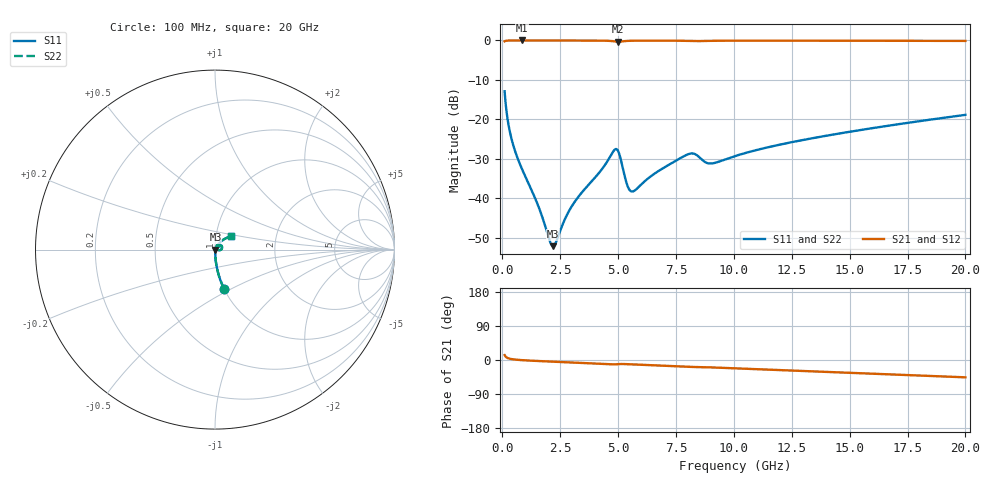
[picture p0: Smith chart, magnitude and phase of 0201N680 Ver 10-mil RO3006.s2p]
# GHz S MA R 50
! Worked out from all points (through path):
!   1601 points, 100 MHz to 20 GHz, reference 50 ohm
!   highest |S21| = -0.02 dB at 833.8 MHz (marker M1); lowest = -0.3 dB at 4.988 GHz (marker M2)
!   group delay of S21, straight-line fit = 6.5 ps
!   lowest |S11| = -52.1 dB at 2.189 GHz (marker M3), VSWR 1.00, Z = 50.2 - j0.0379 ohm
!   |S11| at or under -10 dB: start of sweep to end of sweep
!   |S22| runs from -52.1 to -12.9 dB; largest |S21 - S12| = 0
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0.1  0.2269 -76.9  0.973 12.9  0.973 12.9  0.2269 -76.9
0.274125  0.0836 -85.1  0.9955 4.2  0.9955 4.2  0.0836 -85.1
0.3860625  0.05859 -86.4  0.9972 2.6  0.9972 2.6  0.05859 -86.4
0.8338125  0.02418 -86.7  0.9982 -0.3  0.9982 -0.3  0.02418 -86.7
1.555187  0.008007 -77.8  0.9979 -2.7  0.9979 -2.7  0.008007 -77.8
2.065125  0.00282 -35.7  0.9975 -4.1  0.9975 -4.1  0.00282 -35.7
2.1895  0.002489 -8.7  0.9975 -4.4  0.9975 -4.4  0.002489 -8.7
2.326312  0.002824 19.7  0.9974 -4.8  0.9974 -4.8  0.002824 19.7
2.873562  0.006876 58.4  0.997 -6.2  0.997 -6.2  0.006876 58.4
3.420812  0.01176 65.3  0.9964 -7.5  0.9964 -7.5  0.01176 65.3
4.279  0.02296 64.1  0.9933 -9.9  0.9933 -9.9  0.02296 64.1
4.813813  0.04017 39.8  0.9743 -11.5  0.9743 -11.5  0.04017 39.8
4.987938  0.0405 13.9  0.963 -11.0  0.963 -11.0  0.0405 13.9
5.385937  0.01504 -0.1  0.9851 -11.0  0.9851 -11.0  0.01504 -0.1
5.5725  0.01227 20.9  0.9895 -11.6  0.9895 -11.6  0.01227 20.9
6.741625  0.02219 59.2  0.9935 -14.8  0.9935 -14.8  0.02219 59.2
8.10975  0.03686 47.2  0.9839 -18.2  0.9839 -18.2  0.03686 47.2
8.967937  0.02766 43.1  0.9867 -19.4  0.9867 -19.4  0.02766 43.1
10.05  0.03432 55.6  0.9918 -22.1  0.9918 -22.1  0.03432 55.6
13.37081  0.05765 53.5  0.9914 -29.9  0.9914 -29.9  0.05765 53.5
16.69162  0.08341 47.3  0.9889 -37.8  0.9889 -37.8  0.08341 47.3
20  0.1142 40.2  0.985 -45.7  0.985 -45.7  0.1142 40.2
